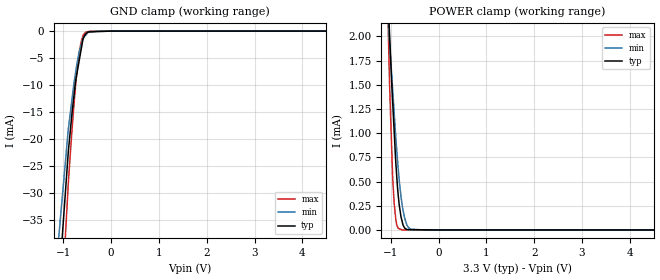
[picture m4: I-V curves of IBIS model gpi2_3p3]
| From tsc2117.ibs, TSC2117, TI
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|   gpi2_3p3 Model
[Model]   gpi2_3p3
Model_type   Input
Vinl = 0.99
Vinh = 2.31
|   typ   min   max
|   (nom PVT)   (fast PVT)   (slow PVT)
|C_comp from frequency sweep method (F=25MHz)
|Average
|C_comp   1.613e-12   1.560e-12   1.641e-12
|C_comp from LC tank measurement(L=1nH)
|Average
|Resonant Frequency(Hz)   5.080e+09   5.110e+09   5.079e+09
C_comp   9.825e-13   9.710e-13   9.829e-13
| Where nom  PVT is Nominal Process, 3.3V, 48C
|   Fast PVT is Strong Process,  3.6V, -40C
|   Slow PVT is Weak Process,   3V, 108C
[Model Spec]
|Subparameter   typ   min   max
Vinh   2.31   2.1   2.52
Vinl   0.99   0.9   1.08
[Voltage Range]   3.3   3   3.6
|Ambient Temperature   25   85   -40
|Junction Temperature
[Temperature Range]   48   108   -40
[Power Clamp Reference]   3.3   3   3.6
[GND Clamp Reference]   0   0   0
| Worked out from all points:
|   GND clamp passes 1 mA (typ) near -0.56 V on its own axis
|   POWER clamp passes 1 mA (typ) near -0.93 V on its own axis
[GND Clamp]
|   Voltage   I(typ)   I(min)   I(max)
-3.3V     -1.744A    -1.584A    -1.955A
-1.498V   -97.24mA   -78.51mA   -125mA
-897.6mV  -22.45mA   -18.25mA   -28.4mA
-788.4mV  -12.73mA   -10.42mA   -14.69mA
-745.8mV  -9.337mA   -7.78mA    -10.25mA
-698.4mV  -6.949mA   -5.254mA   -6.058mA
-622.8mV  -3.141mA   -2.43mA    -1.773mA
-590.7mV  -1.524mA   -1.412mA   -920.3uA
-532.8mV  -547.8uA   -745.6uA   -189.1uA
-474mV    -165.5uA   -162.9uA   -75.95uA
-285mV    -99.09uA   -1.764uA   -4.566uA
6.6V      0A         0A         0A
[POWER Clamp]
|   Voltage   I(typ)   I(min)   I(max)
-3.3V     32.36mA    22.63mA    56.39mA
-1.092V   2.784mA    2.476mA    2.833mA
-1.03V    2.043mA    1.957mA    1.546mA
-964.8mV  1.343mA    1.464mA    567.9uA
-932.4mV  1.031mA    1.218mA    283.9uA
-896.4mV  688.4uA    946.4uA    105.3uA
-858mV    421.1uA    697.5uA    28.3uA
-825mV    257.9uA    511.6uA    12.67uA
-766.8mV  92.84uA    269.4uA    561.8nA
-675mV    8.294uA    64.77uA    317nA
-579mV    3.4uA      6.544uA    221.5nA
6.6V      0A         0A         0A
